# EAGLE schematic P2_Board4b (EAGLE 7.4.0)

## Sheet 1 of 4: Propeller
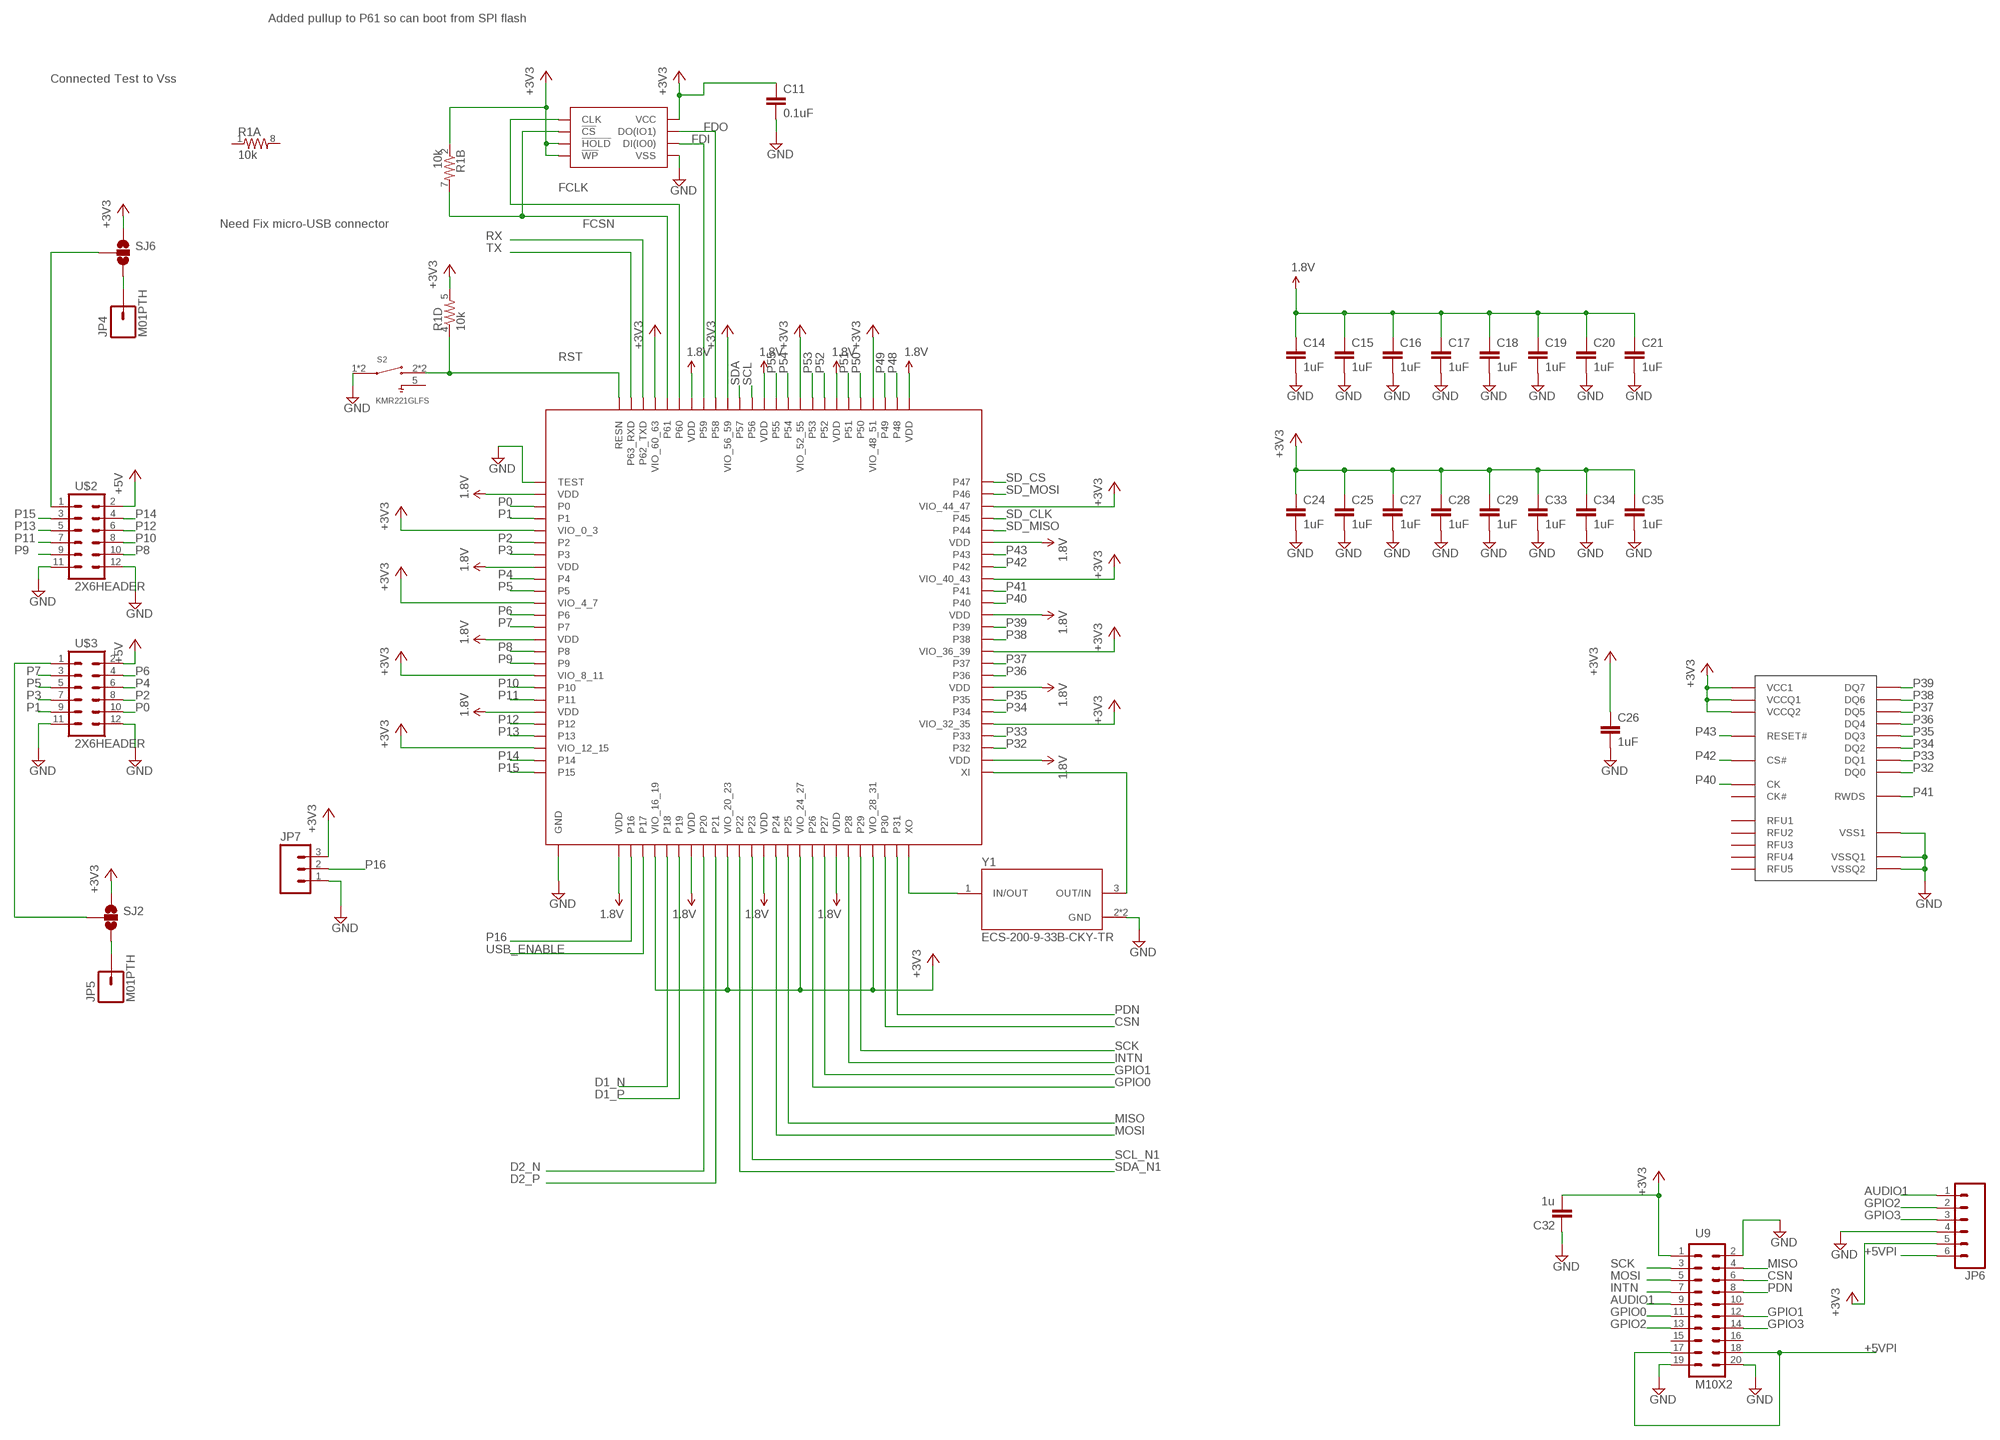
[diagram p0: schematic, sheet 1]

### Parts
C11  0.1uF  1.0UF-25V-+80/-20(0805)  [0805]
C14  1uF  22UF-6.3V-20%(0805)  [0805]
C15  1uF  22UF-6.3V-20%(0805)  [0805]
C16  1uF  22UF-6.3V-20%(0805)  [0805]
C17  1uF  22UF-6.3V-20%(0805)  [0805]
C18  1uF  22UF-6.3V-20%(0805)  [0805]
C19  1uF  22UF-6.3V-20%(0805)  [0805]
C20  1uF  22UF-6.3V-20%(0805)  [0805]
C21  1uF  22UF-6.3V-20%(0805)  [0805]
C24  1uF  22UF-6.3V-20%(0805)  [0805]
C25  1uF  22UF-6.3V-20%(0805)  [0805]
C26  1uF  22UF-6.3V-20%(0805)  [0805]
C27  1uF  22UF-6.3V-20%(0805)  [0805]
C28  1uF  22UF-6.3V-20%(0805)  [0805]
C29  1uF  22UF-6.3V-20%(0805)  [0805]
C32  1u  C-EUC0805  [C0805]
C33  1uF  22UF-6.3V-20%(0805)  [0805]
C34  1uF  22UF-6.3V-20%(0805)  [0805]
C35  1uF  22UF-6.3V-20%(0805)  [0805]
JP4  M01PTH  [1X01]
JP5  M01PTH  [1X01]
JP6  M06LONGPADS  [1X06_LONGPADS]
JP7  M03LONGPADS  [1X03_LONGPADS]
R1  10k  RESISTOR-ARRAY0603-ARV  [0603-ARV]
S2  KMR221GLFS  [SW_KMR221GLFS]
SJ2  SOLDERJUMPER_2WAYPASTE1&2  [SJ_3_PASTE1&2]
SJ6  SOLDERJUMPER_2WAYPASTE1&2  [SJ_3_PASTE1&2]
U2  Propeller 2 - ES  P2X8C4M64P-ES_  [PROPELLER_2]
U3  SPI Flash 16MB (128Mb)  604-10047_:_IC_FLASH_128M_SPI_133MHZ_8SOIC  [SOIC_8_WIDE]
U5  HYPERRAM  [TFBGA24]
U9  M10X2  [2X10]
U$2  2X6HEADER  [6X2HEADER]
U$3  2X6HEADER  [6X2HEADER]
Y1  ECS-200-9-33B-CKY-TR  [XTAL_ECS-200-9-33B-CKY-TR]

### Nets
1.8V: C14.1 C15.1 C16.1 C17.1 C18.1 C19.1 C20.1 C21.1 U2.2(VDD) U2.8(VDD) U2.14(VDD) U2.20(VDD) U2.26(VDD) U2.32(VDD) U2.38(VDD) U2.44(VDD) U2.52(VDD) U2.58(VDD) U2.64(VDD) U2.70(VDD) U2.76(VDD) U2.82(VDD) U2.88(VDD) U2.94(VDD) ; also sheet 4
+3V3: C11.1 C24.1 C25.1 C26.1 C27.1 C28.1 C29.1 C32.2 C33.1 C34.1 C35.1 JP6.5 JP7.3 R1.2 R1.5 SJ2.1 SJ6.1 U2.5(VIO_0_3) U2.11(VIO_4_7) U2.17(VIO_8_11) U2.23(VIO_12_15) U2.29(VIO_16_19) U2.35(VIO_20_23) U2.41(VIO_24_27) U2.47(VIO_28_31) U2.55(VIO_32_35) U2.61(VIO_36_39) U2.67(VIO_40_43) U2.73(VIO_44_47) U2.79(VIO_48_51) U2.85(VIO_52_55) U2.91(VIO_56_59) U2.97(VIO_60_63) U3.3(!WP) U3.7(!HOLD) U3.8(VCC) U5.P$9(VCC1) U5.P$16(VCCQ1) U5.P$24(VCCQ2) U9.1 ; also sheet 3,4
+5V: U$2.2 U$3.2 ; also sheet 2,3,4
+5VPI: JP6.6 U9.17 U9.18 ; also sheet 4
AUDIO1: JP6.1 U9.9
CSN: U2.48(P30) U9.6
D1_N: U2.30(P18) ; also sheet 3
D1_P: U2.31(P19) ; also sheet 3
D2_N: U2.33(P20) ; also sheet 3
D2_P: U2.34(P21) ; also sheet 3
FCLK: U2.95(P60) U3.6(CLK)
FCSN: R1.7 U2.96(P61) U3.1(!CS)
FDI: U2.93(P59) U3.5(DI(IO0))
FDO: U2.92(P58) U3.2(DO(IO1))
GND [power]: C11.2 C14.2 C15.2 C16.2 C17.2 C18.2 C19.2 C20.2 C21.2 C24.2 C25.2 C26.2 C27.2 C28.2 C29.2 C32.1 C33.2 C34.2 C35.2 JP6.4 JP7.1 S2.1 S2.4 U2.1(TEST) U2.EP(GND) U3.4(VSS) U5.P$8(VSS1) U5.P$11(VSSQ1) U5.P$25(VSSQ2) U9.2 U9.19 U9.20 U$2.11 U$2.12 U$3.11 U$3.12 Y1.2(GND) Y1.4(GND) ; also sheet 2,3,4
GPIO0: U2.42(P26) U9.11
GPIO1: U2.43(P27) U9.12
GPIO2: JP6.2 U9.13
GPIO3: JP6.3 U9.14
INTN: U2.45(P28) U9.7
MISO: U2.40(P25) U9.4
MOSI: U2.39(P24) U9.5
N$1: U2.51(XI) Y1.3(OUT/IN)
N$3: U2.50(XO) Y1.1(IN/OUT)
N$10: SJ6.2 U$2.1
N$14: JP4.1 SJ6.3
N$32: SJ2.2 U$3.1
N$33: JP5.1 SJ2.3
P0: U2.3(P0) U$3.10
P1: U2.4(P1) U$3.9
P2: U2.6(P2) U$3.8
P3: U2.7(P3) U$3.7
P4: U2.9(P4) U$3.6
P5: U2.10(P5) U$3.5
P6: U2.12(P6) U$3.4
P7: U2.13(P7) U$3.3
P8: U2.15(P8) U$2.10
P9: U2.16(P9) U$2.9
P10: U2.18(P10) U$2.8
P11: U2.19(P11) U$2.7
P12: U2.21(P12) U$2.6
P13: U2.22(P13) U$2.5
P14: U2.24(P14) U$2.4
P15: U2.25(P15) U$2.3
P16: JP7.2 U2.27(P16) ; also sheet 3
P32: U2.53(P32) U5.P$18(DQ0)
P33: U2.54(P33) U5.P$17(DQ1)
P34: U2.56(P34) U5.P$14(DQ2)
P35: U2.57(P35) U5.P$19(DQ3)
P36: U2.59(P36) U5.P$20(DQ4)
P37: U2.60(P37) U5.P$23(DQ5)
P38: U2.62(P38) U5.P$22(DQ6)
P39: U2.63(P39) U5.P$21(DQ7)
P40: U2.65(P40) U5.P$7(CK)
P41: U2.66(P41) U5.P$13(RWDS)
P42: U2.68(P42) U5.P$3(CS#)
P43: U2.69(P43) U5.P$4(RESET#)
P48: U2.77(P48) ; also sheet 3
P49: U2.78(P49) ; also sheet 3
P50: U2.80(P50) ; also sheet 3
P51: U2.81(P51) ; also sheet 3
P52: U2.83(P52) ; also sheet 3
P53: U2.84(P53) ; also sheet 3
P54: U2.86(P54) ; also sheet 3
P55: U2.87(P55) ; also sheet 3
PDN: U2.49(P31) U9.8
RST: R1.4 S2.2 S2.3 U2.100(RESN) ; also sheet 2,4
RX: U2.98(P62_TXD) ; also sheet 2
SCK: U2.46(P29) U9.3
SCL: U2.89(P56) ; also sheet 3
SCL_N1: U2.37(P23) ; also sheet 3
SD_CLK: U2.72(P45) ; also sheet 3
SD_CS: U2.75(P47) ; also sheet 3
SD_MISO: U2.71(P44) ; also sheet 3
SD_MOSI: U2.74(P46) ; also sheet 3
SDA: U2.90(P57) ; also sheet 3
SDA_N1: U2.36(P22) ; also sheet 3
TX: U2.99(P63_RXD) ; also sheet 2
USB_ENABLE: U2.28(P17) ; also sheet 3
Unconnected: R1.1 R1.8 S2.5 U5.P$2(RFU1) U5.P$5(RFU2) U5.P$6(CK#) U5.P$10(RFU3) U5.P$12(RFU4) U5.P$15(RFU5) U9.10 U9.15 U9.16

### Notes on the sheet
- Added pullup to P61 so can boot from SPI flash
- Connected Test to Vss
- Need Fix micro-USB connector

## Sheet 2 of 4: FT231X
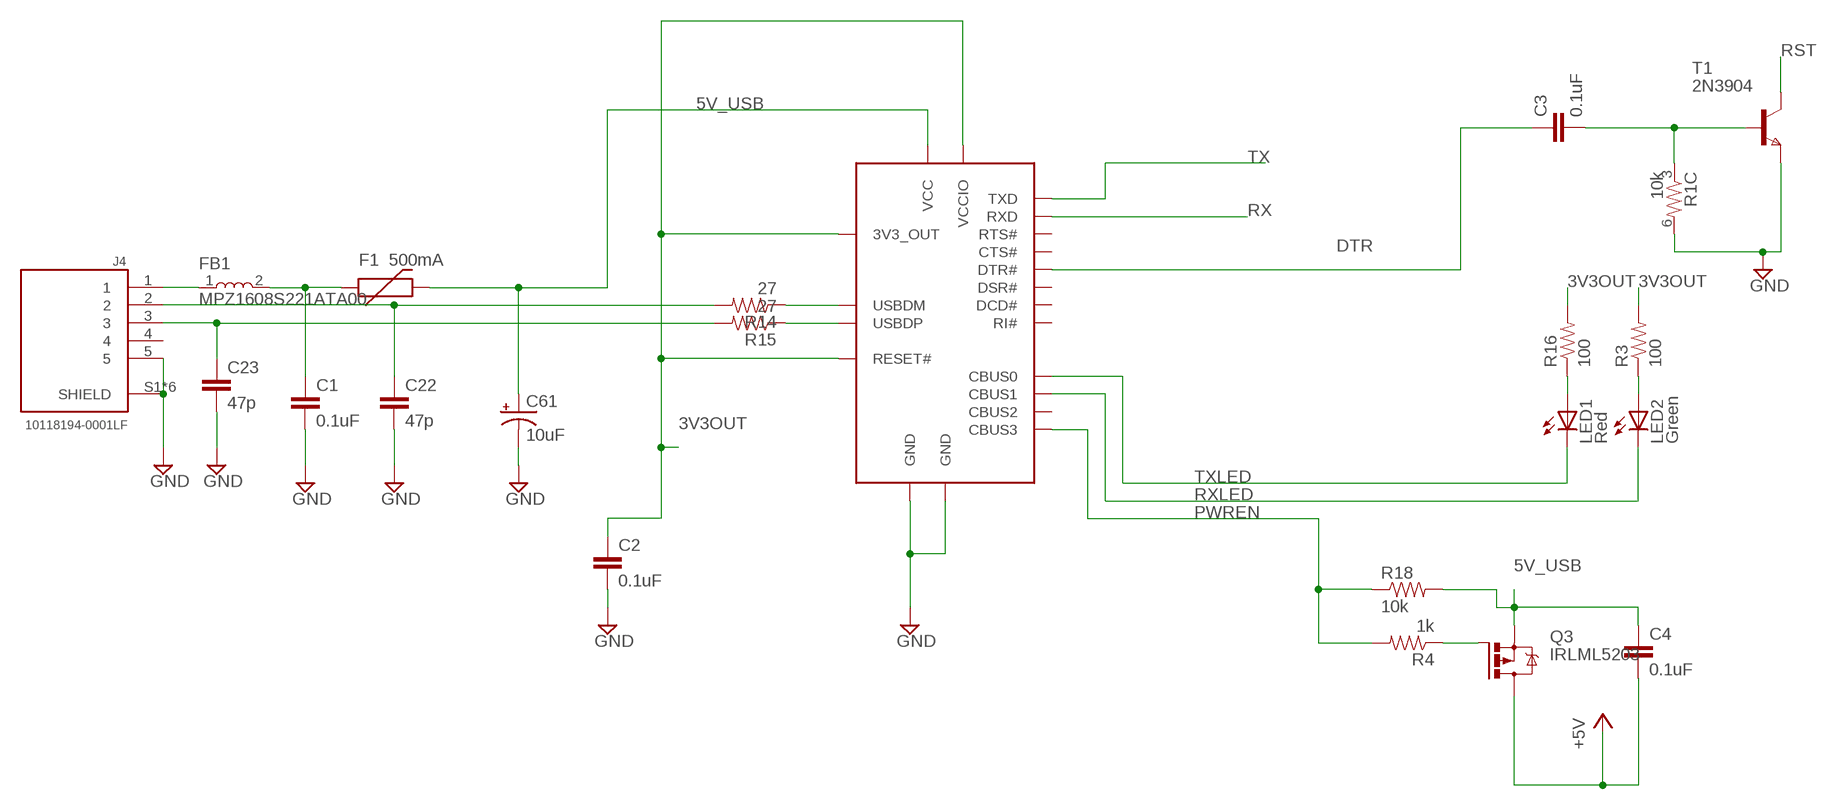
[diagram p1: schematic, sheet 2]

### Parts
C1  0.1uF  1.0UF-25V-+80/-20(0805)  [0805]
C2  0.1uF  1.0UF-25V-+80/-20(0805)  [0805]
C3  0.1uF  1.0UF-25V-+80/-20(0805)  [0805]
C4  0.1uF  1.0UF-25V-+80/-20(0805)  [0805]
C22  47p  1.0UF-25V-+80/-20(0805)  [0805]
C23  47p  1.0UF-25V-+80/-20(0805)  [0805]
C61  10uF  CAP_POL1206  [EIA3216]
F1  500mA  PTCSMD  [PTC-1206]
FB1  MPZ1608S221ATA00  [INDC1608X80]
J4  10118194-0001LF  [AMPHENOL_10118194-0001LF]
LED1  Red  LEDSML0805  [SML0805]
LED2  Green  LEDSML0805  [SML0805]
Q3  IRLML5203  [MICRO3]
R3  100  0.75OHM1/4W1%(0805)  [0805]
R4  1k  0.75OHM1/4W1%(0805)  [0805]
R14  27  0.75OHM1/4W1%(0805)  [0805]
R15  27  0.75OHM1/4W1%(0805)  [0805]
R16  100  0.75OHM1/4W1%(0805)  [0805]
R18  10k  0.75OHM1/4W1%(0805)  [0805]
T1  2N3904  NPNSOT23  [SOT-23]
U1  FT231XS-R  604-00065_:_IC-FTDI,_FT231X  [SSOP20]

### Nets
3V3OUT [power]: C2.1 R3.2 R16.2 U1.3(VCCIO) U1.13(3V3_OUT) U1.14(RESET#)
5V_USB [power]: C4.1 C61.A(+) F1.2 Q3.2(S) R18.2 U1.15(VCC)
+5V: C4.2 Q3.3(D) ; also sheet 1,3,4
DTR: C3.1 U1.1(DTR#)
GND [power]: C1.2 C2.2 C22.2 C23.2 C61.C(-) J4.5 J4.S1(SHIELD) J4.S2(SHIELD) J4.S3(SHIELD) J4.S4(SHIELD) J4.S5(SHIELD) J4.S6(SHIELD) R1.6 T1.2(E) U1.6(GND) U1.16(GND) ; also sheet 1,3,4
N$2: LED1.A R16.1
N$8: FB1.1 J4.1
N$9: C1.1 F1.1 FB1.2
N$11: R14.1 U1.12(USBDM)
N$12: R15.1 U1.11(USBDP)
N$15: C22.1 J4.2 R14.2
N$16: C23.1 J4.3 R15.2
N$18: LED2.A R3.1
N$24: Q3.1(G) R4.1
N$25: C3.2 R1.3 T1.3(B)
PWREN: R4.2 R18.1 U1.19(CBUS3)
RST: T1.1(C) ; also sheet 1,4
RX: U1.4(RXD) ; also sheet 1
RXLED: LED2.C U1.17(CBUS1)
TX: U1.20(TXD) ; also sheet 1
TXLED: LED1.C U1.18(CBUS0)
Unconnected: J4.4 U1.2(RTS#) U1.5(RI#) U1.7(DSR#) U1.8(DCD#) U1.9(CTS#) U1.10(CBUS2)

## Sheet 3 of 4: Wings
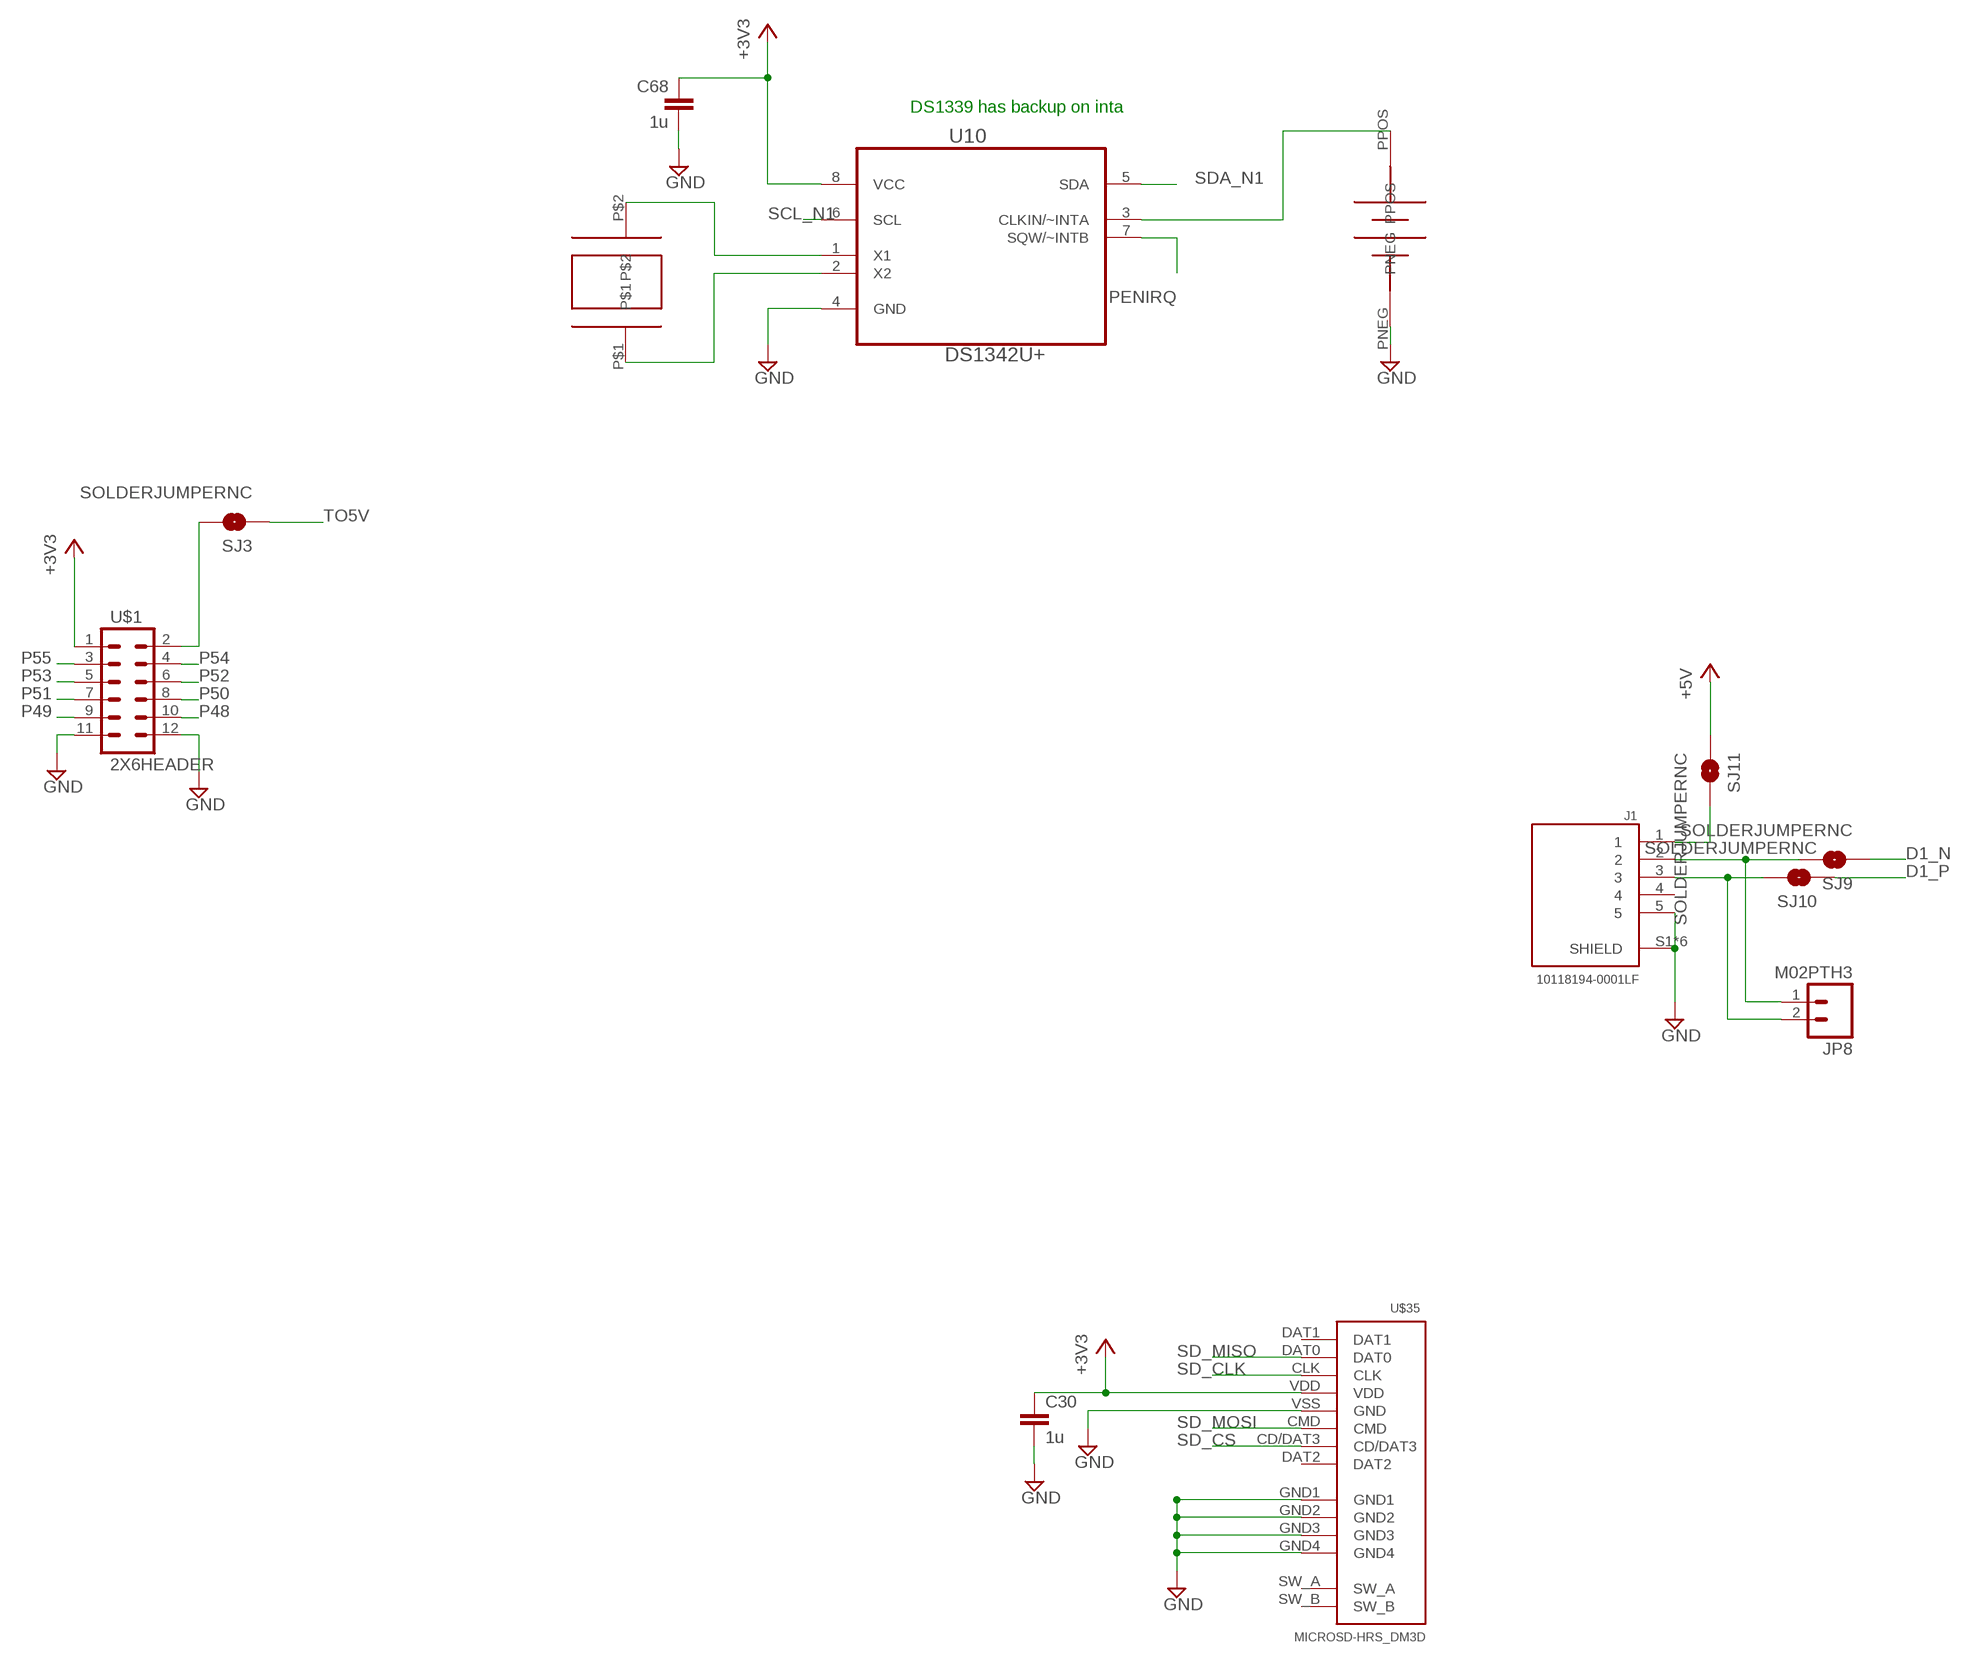
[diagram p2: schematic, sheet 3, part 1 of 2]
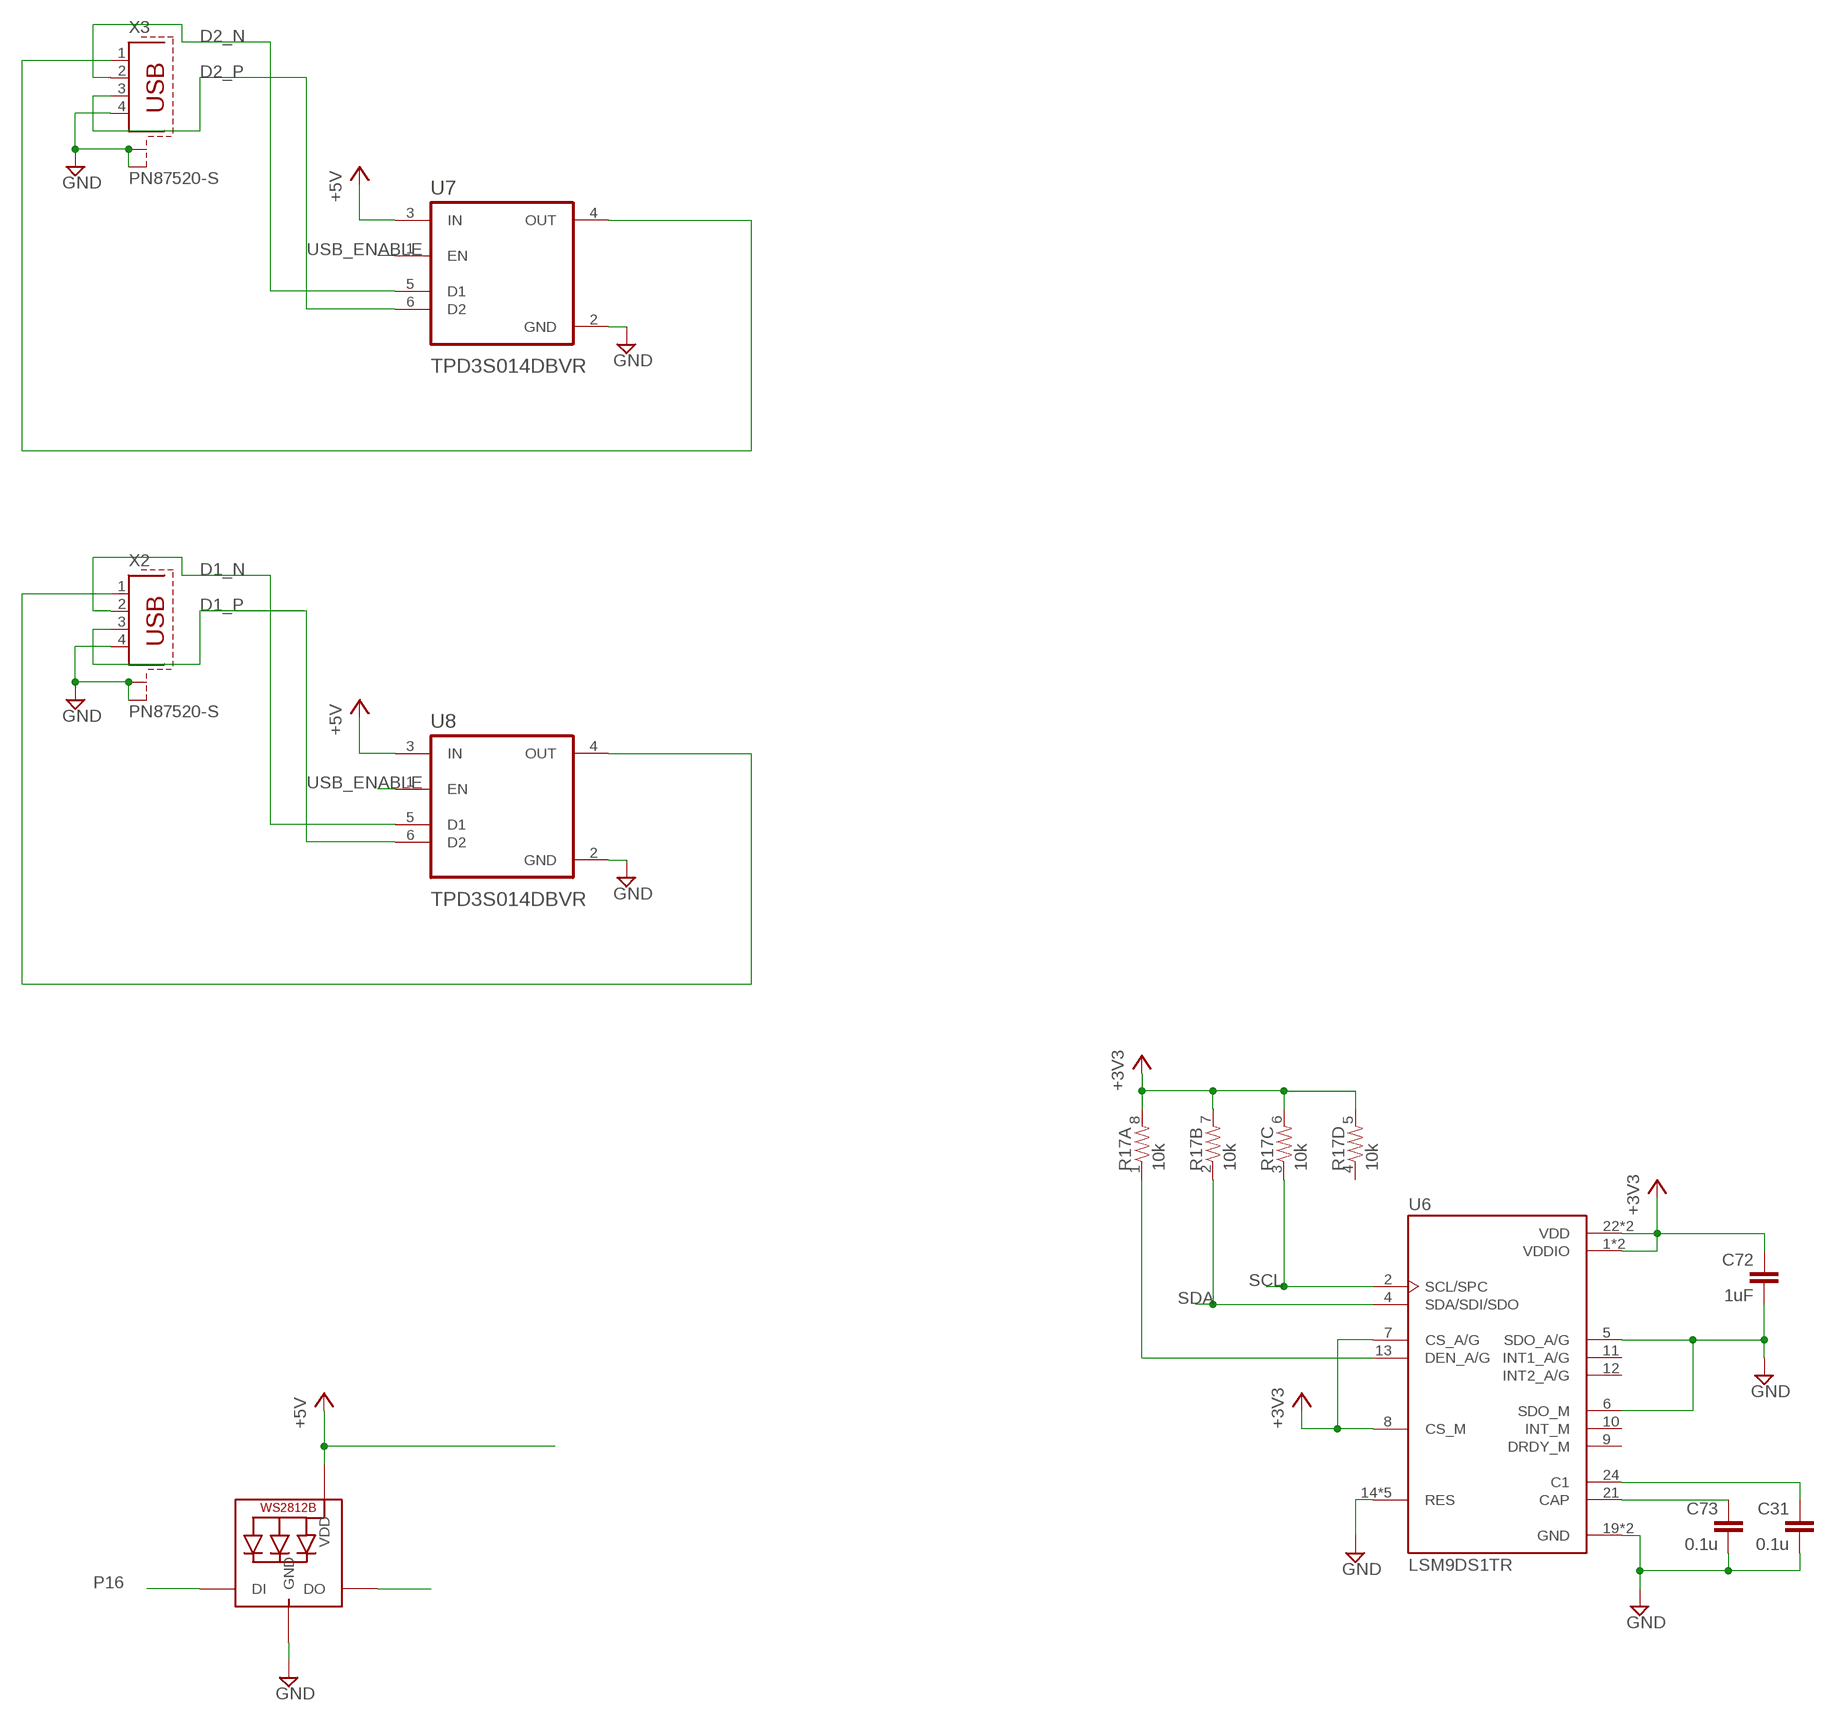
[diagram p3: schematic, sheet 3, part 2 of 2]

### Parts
C30  1u  C-EUC0805  [C0805]
C31  0.1u  4.7UF-6.3V-10%(0603)0603  [0603-CAP]
C68  1u  4.7UF-6.3V-10%(0603)0603  [0603-CAP]
C71  RAY2_SUPERCAP  [RAY2_SUPERCAP]
C72  1uF  4.7UF-6.3V-10%(0603)0603  [0603-CAP]
C73  0.1u  4.7UF-6.3V-10%(0603)0603  [0603-CAP]
J1  10118194-0001LF  [AMPHENOL_10118194-0001LF]
JP8  M02PTH3  [1X02_LONGPADS]
LED3  WS2812B3535  [LED3535]
R17  10k  RESISTOR-ARRAY0603-ARV  [0603-ARV]
SJ3  SOLDERJUMPERNC  [SJ_2S]
SJ9  SOLDERJUMPERNC  [SJ_2S]
SJ10  SOLDERJUMPERNC  [SJ_2S]
SJ11  SOLDERJUMPERNC  [SJ_2S]
U6  LSM9DS1TR  [PQFN43P300X350X102-24N]
U7  TPD3S014DBVR  [SOT95P280X145-6N]
U8  TPD3S014DBVR  [SOT95P280X145-6N]
U10  DS1342U+  [SOP65P490X110-8N]
U$1  2X6HEADER  [6X2HEADER]
U$35  MICROSD-HRS_DM3D  [DM3D]
X2  PN87520-S  [PN87520-S]
X3  PN87520-S  [PN87520-S]
X5  RAY2_SMT_CRYSTAL  [RAY2_SMT_CRYSTAL]

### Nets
+3V3: C30.1 C68.1 C72.1 R17.5 R17.6 R17.7 R17.8 U6.1(VDDIO) U6.3(VDDIO) U6.7(CS_A/G) U6.8(CS_M) U6.22(VDD) U6.23(VDD) U10.8(VCC) U$1.1 U$35.VDD ; also sheet 1,4
+5V: LED3.2(VDD) SJ11.1 U7.3(IN) U8.3(IN) ; also sheet 1,2,4
D1_N: SJ9.1 U8.5(D1) X2.2 ; also sheet 1
D1_P: SJ10.1 U8.6(D2) X2.3 ; also sheet 1
D2_N: U7.5(D1) X3.2 ; also sheet 1
D2_P: U7.6(D2) X3.3 ; also sheet 1
GND [power]: C30.2 C31.2 C68.2 C71.PNEG C72.2 C73.2 J1.5 J1.S1(SHIELD) J1.S2(SHIELD) J1.S3(SHIELD) J1.S4(SHIELD) J1.S5(SHIELD) J1.S6(SHIELD) LED3.4(GND) U6.5(SDO_A/G) U6.6(SDO_M) U6.14(RES) U6.15(RES) U6.16(RES) U6.17(RES) U6.18(RES) U6.19(GND) U6.20(GND) U7.2(GND) U8.2(GND) U10.4(GND) U$1.11 U$1.12 U$35.GND1 U$35.GND2 U$35.GND3 U$35.GND4 U$35.VSS(GND) X2.4 X2.S1 X2.S2 X3.4 X3.S1 X3.S2 ; also sheet 1,2,4
N$17: U7.4(OUT) X3.1
N$28: U8.4(OUT) X2.1
N$29: C73.1 U6.21(CAP)
N$30: C31.1 U6.24(C1)
N$31: R17.1 U6.13(DEN_A/G)
N$39: LED3.3(DO)
N$40: J1.2 JP8.1 SJ9.2
N$41: J1.3 JP8.2 SJ10.2
N$42: J1.1 SJ11.2
N$43: SJ3.2 U$1.2
N$78: C71.PPOS U10.3(CLKIN/~INTA)
N$79: U10.2(X2) X5.P$1
N$81: U10.1(X1) X5.P$2
P16: LED3.1(DI) ; also sheet 1
P48: U$1.10 ; also sheet 1
P49: U$1.9 ; also sheet 1
P50: U$1.8 ; also sheet 1
P51: U$1.7 ; also sheet 1
P52: U$1.6 ; also sheet 1
P53: U$1.5 ; also sheet 1
P54: U$1.4 ; also sheet 1
P55: U$1.3 ; also sheet 1
PENIRQ: U10.7(SQW/~INTB)
SCL: R17.3 U6.2(SCL/SPC) ; also sheet 1
SCL_N1: U10.6(SCL) ; also sheet 1
SD_CLK: U$35.CLK ; also sheet 1
SD_CS: U$35.CD/DAT3 ; also sheet 1
SD_MISO: U$35.DAT0 ; also sheet 1
SD_MOSI: U$35.CMD ; also sheet 1
SDA: R17.2 U6.4(SDA/SDI/SDO) ; also sheet 1
SDA_N1: U10.5(SDA) ; also sheet 1
TO5V: SJ3.1 ; also sheet 4
USB_ENABLE: U7.1(EN) U8.1(EN) ; also sheet 1
Unconnected: J1.4 R17.4 U6.9(DRDY_M) U6.10(INT_M) U6.11(INT1_A/G) U6.12(INT2_A/G) U$35.DAT1 U$35.DAT2 U$35.SW_A U$35.SW_B

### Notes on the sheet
- DS1339 has backup on inta

## Sheet 4 of 4: Power
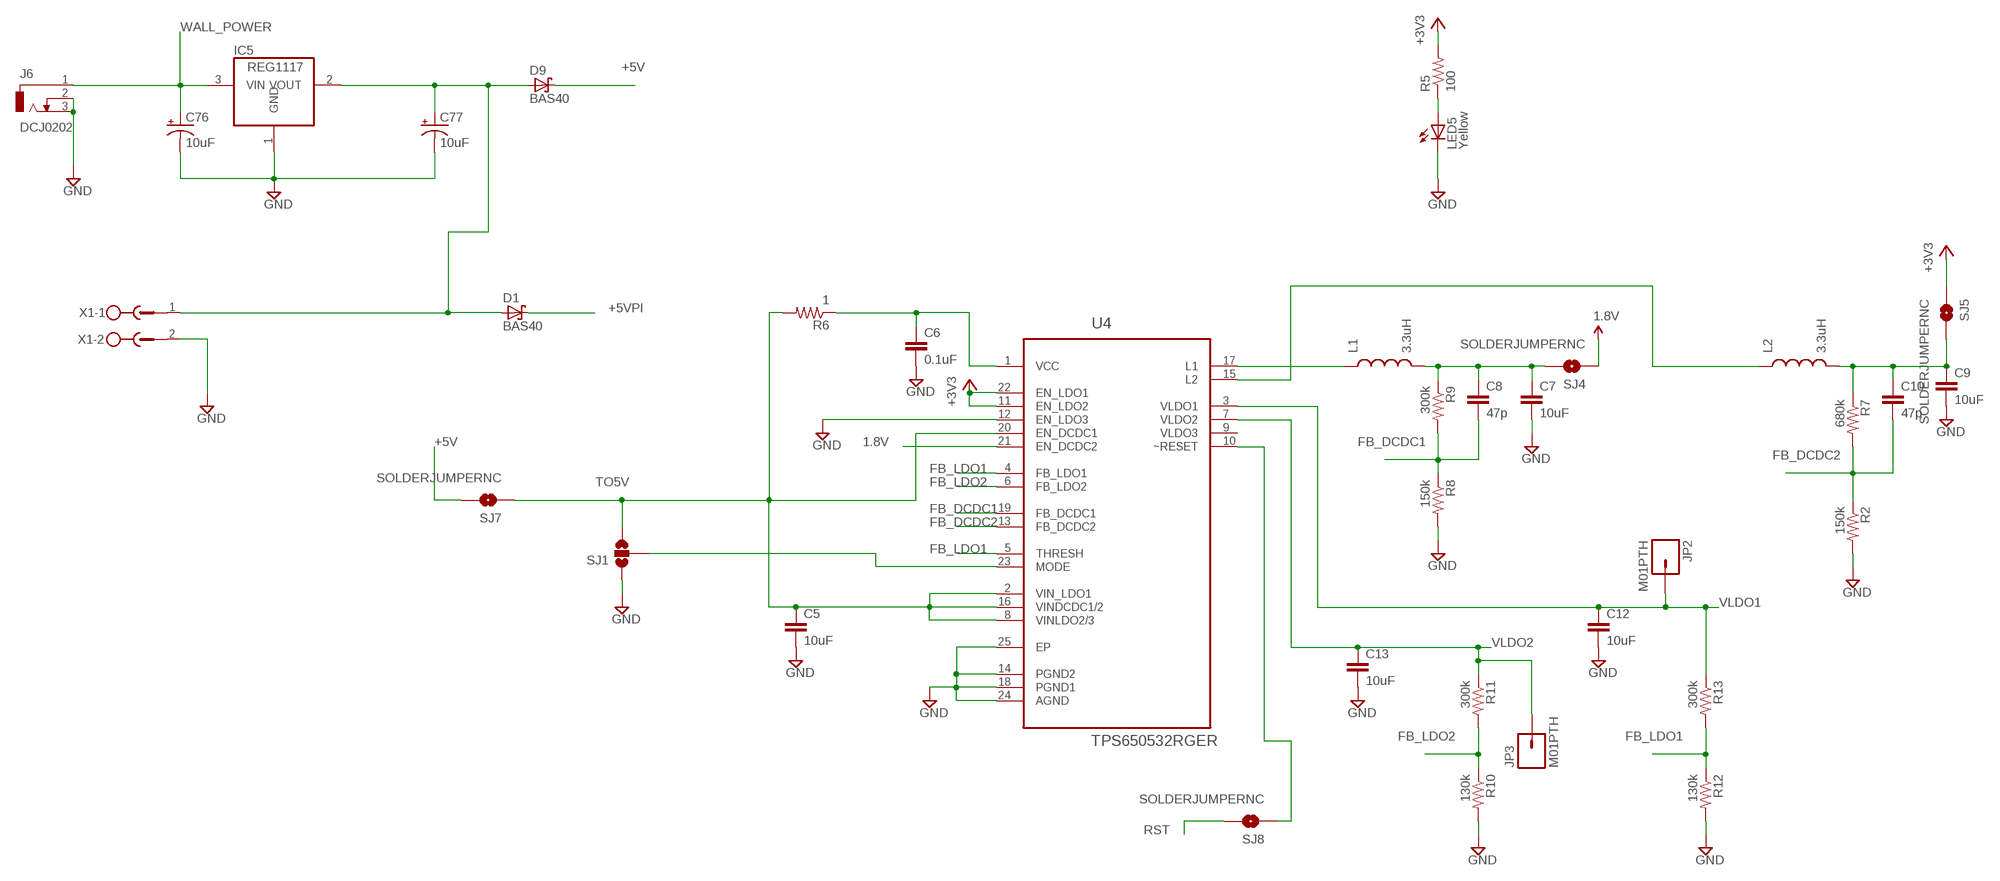
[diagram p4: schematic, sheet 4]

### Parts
C5  10uF  22UF-6.3V-20%(0805)  [0805]
C6  0.1uF  1.0UF-25V-+80/-20(0805)  [0805]
C7  10uF  22UF-6.3V-20%(0805)  [0805]
C8  47p  1.0UF-25V-+80/-20(0805)  [0805]
C9  10uF  22UF-6.3V-20%(0805)  [0805]
C10  47p  1.0UF-25V-+80/-20(0805)  [0805]
C12  10uF  22UF-6.3V-20%(0805)  [0805]
C13  10uF  22UF-6.3V-20%(0805)  [0805]
C76  10uF  10UF-16V-10%(TANT)  [EIA3216]
C77  10uF  10UF-16V-10%(TANT)  [EIA3216]
D1  BAS40  [SOT23]
D9  BAS40  [SOT23]
IC5  REG1117  [SOT223]
J6  DCJ0202  [DCJ0202]
JP2  M01PTH  [1X01]
JP3  M01PTH  [1X01]
L1  3.3uH  INDUCTOR1210  [1210]
L2  3.3uH  INDUCTOR1210  [1210]
LED5  Yellow  LEDSML0805  [SML0805]
R2  150k  0.75OHM1/4W1%(0805)  [0805]
R5  100  0.75OHM1/4W1%(0805)  [0805]
R6  1  0.75OHM1/4W1%(0805)  [0805]
R7  680k  0.75OHM1/4W1%(0805)  [0805]
R8  150k  0.75OHM1/4W1%(0805)  [0805]
R9  300k  0.75OHM1/4W1%(0805)  [0805]
R10  130k  0.75OHM1/4W1%(0805)  [0805]
R11  300k  0.75OHM1/4W1%(0805)  [0805]
R12  130k  0.75OHM1/4W1%(0805)  [0805]
R13  300k  0.75OHM1/4W1%(0805)  [0805]
SJ1  SOLDERJUMPER_2WAYPASTE1&2  [SJ_3_PASTE1&2]
SJ4  SOLDERJUMPERNC  [SJ_2S]
SJ5  SOLDERJUMPERNC  [SJ_2S]
SJ7  SOLDERJUMPERNC  [SJ_2S]
SJ8  SOLDERJUMPERNC  [SJ_2S]
U4  TPS650532RGER  [QFN50P400X400X100-25N]
X1  MSTBV2  [MSTBV2]

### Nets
1.8V: SJ4.1 U4.21(EN_DCDC2) ; also sheet 1
+3V3: R5.2 SJ5.1 U4.11(EN_LDO2) U4.22(EN_LDO1) ; also sheet 1,3
+5_VIN: C77.A(+) D1.1(A) D9.1(A) IC5.2(VOUT) X1.1
+5V: D9.3(C) SJ7.2 ; also sheet 1,2,3
+5VPI: D1.3(C) ; also sheet 1
FB_DCDC1: C8.2 R8.1 R9.2 U4.19(FB_DCDC1)
FB_DCDC2: C10.2 R2.1 R7.2 U4.13(FB_DCDC2)
FB_LDO1: R12.1 R13.2 U4.4(FB_LDO1) U4.5(THRESH)
FB_LDO2: R10.1 R11.2 U4.6(FB_LDO2)
GND [power]: C5.2 C6.2 C7.2 C9.2 C12.2 C13.2 C76.C(-) C77.C(-) IC5.1(GND) J6.2 J6.3 LED5.C R2.2 R8.2 R10.2 R12.2 SJ1.1 U4.12(EN_LDO3) U4.14(PGND2) U4.18(PGND1) U4.24(AGND) U4.25(EP) X1.2 ; also sheet 1,2,3
N$4: L2.1 U4.15(L2)
N$5: SJ1.2 U4.23(MODE)
N$6: C6.1 R6.1 U4.1(VCC)
N$7: L1.1 U4.17(L1)
N$13: SJ8.1 U4.10(~RESET)
N$22: C7.1 C8.1 L1.2 R9.1 SJ4.2
N$34: C9.1 C10.1 L2.2 R7.1 SJ5.2
N$45: LED5.A R5.1
RST: SJ8.2 ; also sheet 1,2
TO5V: C5.1 R6.2 SJ1.3 SJ7.1 U4.2(VIN_LDO1) U4.8(VINLDO2/3) U4.16(VINDCDC1/2) U4.20(EN_DCDC1) ; also sheet 3
VLDO1: C12.1 JP2.1 R13.1 U4.3(VLDO1)
VLDO2: C13.1 JP3.1 R11.1 U4.7(VLDO2)
WALL_POWER: C76.A(+) IC5.3(VIN) J6.1
Unconnected: U4.9(VLDO3)

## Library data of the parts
C1-C4 C6 C8 C10 C11 C22 C23 = SparkFun-Capacitors:1.0UF-25V-+80/-20(0805); PROD_ID: CAP-11625; VALUE: 1.0uF
C5 C7 C9 C12-C21 C24-C29 C33-C35 = SparkFun-Capacitors:22UF-6.3V-20%(0805): Ceramic; PROD_ID: CAP-08402; VALUE: 22uF
C30 C32 = rcl:C-EU: CAPACITOR, European symbol
C31 C68 C72 C73 = SparkFun-Capacitors:4.7UF-6.3V-10%(0603): CAP-08280; PROD_ID: CAP-08280; VALUE: 4.7uF
C61 = SparkFun:CAP_POL: Capacitor Polarized
C71 = Manta1:RAY2_SUPERCAP
C76 C77 = SparkFun-Capacitors:10UF-16V-10%(TANT): CAP-00811; PROD_ID: CAP-00811
D1 D9 = diode:BAS40: Silicon Schottky Diodes
F1 = SparkFun:PTC: Resettable Fuse PTC
FB1 = ray2:MPZ1608S221ATA00: Ind Chip Bead Multi-Layer 220Ohm 25% 100MHz Ferrite 2.2A 0603 Punched Paper T/R; DESCRIPTION: Ind Chip Bead Multi-Layer 220Ohm 25% 100MHz Ferrite 2.2A 0603 Punched Paper T/R; DIGI-KEY_PART_NUMBER: 445-1565-1-ND; DIGI-KEY_PURCHASE_URL: https://www.digikey.com/product-detail/en/tdk-corporation/MPZ1608S221ATA00/445-1565-1-ND/571895?utm_source=snapeda&utm_medium=aggregator&utm_campaign=symbol; MF: TDK; MP: MPZ1608S221ATA00; PACKAGE: 0603 TDK
IC5 = burr-brown:REG1117: 800mA and 1A Low Dropout (LDO) Positive Regulator 1.8V, 2.5V, 2.85V, 3.3V, 5V, and Adj; MPN: REG1117; OC_FARNELL: 1097566; OC_NEWARK: 14P6981
J1 J4 = ray2:10118194-0001LF: Micro Usb, 2.0 Type b, Rcpt, Smt; DESCRIPTION: Micro Usb, 2.0 Type b, Rcpt, Smt; DIGI-KEY_PART_NUMBER: 609-4618-1-ND; DIGI-KEY_PURCHASE_URL: https://www.digikey.com/product-detail/en/amphenol-icc-fci/10118194-0001LF/609-4618-1-ND/2785382?utm_source=snapeda&utm_medium=aggregator&utm_campaign=symbol; MF: Amphenol ICC; MP: 10118194-0001LF; PACKAGE: None
J6 = con-jack:DCJ0202: DC POWER JACK Source: DCJ0202.pdf; OC_FARNELL: unknown; OC_NEWARK: unknown
JP2-JP5 = SparkFun-Connectors:M01: Header 1
JP6 = SparkFun-Connectors:M06: Header 6 Standard 6-pin 0.1" header. Use with straight break away headers (SKU : PRT-00116), right angle break away headers (PRT-00553), swiss pins (PRT-00743), machine pins (PRT-00117), and female headers (PRT-00115). Molex polarized connector foot print use with SKU : PRT-08094 with associated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
JP7 = SparkFun-Connectors:M03: Header 3 Standard 3-pin 0.1" header. Use with straight break away headers (SKU : PRT-00116), right angle break away headers (PRT-00553), swiss pins (PRT-00743), machine pins (PRT-00117), and female headers (PRT-00115). Molex polarized connector foot print use with SKU : PRT-08232 with associated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
JP8 = SparkFun-Connectors:M02: Standard 2-pin 0.1" header. Use with
L1 L2 = SparkFun-Passives:INDUCTOR: Inductors
LED1 LED2 LED5 = led:LED: LED
LED3 = adafruit:WS2812B
Q3 = transistor-power:IRLML5203: HEXFET P-Channel Power MOSFET
R1 R17 = SparkFun-Passives:RESISTOR-ARRAY: Array Chip Resistor Source: RS Component / Phycomp
R2-R16 R18 = SparkFun-Resistors:0.75OHM1/4W1%(0805): RES-08474; PROD_ID: RES-08474; VALUE: 0.75
S2 = ray2:KMR221GLFS: Switch Tactile N.O. SPST Button Gull Wing 0.05A 32VDC 1VA 200000Cycles 2N SMD Automotive T/R; DESCRIPTION: Switch Tactile N.O. SPST Button Gull Wing 0.05A 32VDC 1VA 200000Cycles 2N SMD Automotive T/R; DIGI-KEY_PART_NUMBER: 401-1427-1-ND; DIGI-KEY_PURCHASE_URL: https://www.digikey.com/product-detail/en/c-k/KMR221GLFS/401-1427-1-ND/550466?utm_source=snapeda&utm_medium=aggregator&utm_campaign=symbol; MF: C&K; MP: KMR221GLFS; PACKAGE: None
SJ1 SJ2 SJ6 = SparkFun-Passives:SOLDERJUMPER_2WAY: Solder Jumper 2 way solder jumper
SJ3-SJ5 SJ7-SJ11 = SparkFun-Passives:SOLDERJUMPER: Solder Jumper
T1 = zetex:NPNSOT23: NPN TRANSISTOR; MPN: DSS20201L-7; OC_FARNELL: 1710688; OC_NEWARK: 25R4555
U1 = ray2:604-00065_:_IC-FTDI,_FT231X; MANUFACTURER: FTDI : FT231XS-R; POPULATED: True
U2 = ray2:P2X8C4M64P-ES_; MANUFACTURER: Parallax : P2X8C4M64P-ES
U3 = ray2:604-10047_:_IC_FLASH_128M_SPI_133MHZ_8SOIC; MANUFACTURER: Winbond : W25Q128JVSIM TR
U4 = ray2:TPS650532RGER: 5-CHANNEL POWER MGMT IC WITH TWO STEP DOWN CONVERTERS; DESCRIPTION: 5-Channel Power Management IC _PMIC_ with two step down converters and 3 low-input voltage LDOs 24-VQFN -40 to 85; DIGI-KEY_PART_NUMBER: 296-25183-1-ND; DIGI-KEY_PURCHASE_URL: https://www.digikey.com/product-detail/en/texas-instruments/TPS650532RGER/296-25183-1-ND/2171110?utm_source=snapeda&utm_medium=aggregator&utm_campaign=symbol; MF: Texas Instruments; MP: TPS650532RGER; PACKAGE: VQFN-24 Texas Instruments
U5 = ray2:HYPERRAM: ISSI HyperRAM with 24-ball BGA
U6 = ray2:LSM9DS1TR: The LSM9DS1 is a system-in-package featuring a 3D digital linear acceleration sensor, a 3D digital angular rate sensor, and a 3D digital magnetic sensor.; DESCRIPTION: LSM9DS1 Series ±2/±4/±8/±16 g 3D Digital Linear Acceleration Sensor - LGA-24; DIGI-KEY_PART_NUMBER: 497-14946-1-ND; DIGI-KEY_PURCHASE_URL: https://www.digikey.com/product-detail/en/stmicroelectronics/LSM9DS1TR/497-14946-1-ND/4988079?utm_source=snapeda&utm_medium=aggregator&utm_campaign=symbol; MF: STMicroelectronics; MP: LSM9DS1TR; PACKAGE: TFLGA-24 STMicroelectronics
U7 U8 = ray2:TPD3S014DBVR: Current Limit Switch and D+/D? ESD Protection for USB Host Ports 6-SOT-23 -40 to 85; DESCRIPTION: Current Limit Switch and D+/D? ESD Protection for USB Host Ports 6-SOT-23 -40 to 85; DIGI-KEY_PART_NUMBER: 296-38835-1-ND; DIGI-KEY_PURCHASE_URL: https://www.digikey.com/product-detail/en/texas-instruments/TPD3S014DBVR/296-38835-1-ND/5138398?utm_source=snapeda&utm_medium=aggregator&utm_campaign=symbol; MF: Texas Instruments; MP: TPD3S014DBVR; PACKAGE: SOT-23-6 Texas Instruments
U9 = SparkFun-Connectors:M10X2: This was SPECIALLY designed to be used with our Graphic LCD Backpack. Be sure you want to use this! It is not only staggered on each line of header holes, but IT IS ALSO offset of the center point of the top and bottom lines by 5 mil. This causes the headers to lock into place on the "standard"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
U10 = Maxim_By_element14_Batch_1:DS1342U+: Low-Current I2C RTCs for High-ESR Crystals; MPN: DS1342U+; OC_FARNELL: -; OC_NEWARK: 68R0491; PACKAGE: SOP-8; SUPPLIER: Maxim
U$1-U$3 = ray2:2X6HEADER
U$35 = hrs_DM3D-SF:MICROSD-HRS_DM3D
X1 = con-phoenix-500:MSTBV2: PHOENIX; OC_FARNELL: unknown; OC_NEWARK: unknown
X2 X3 = con-berg:PN87520-S; OC_FARNELL: unknown; OC_NEWARK: unknown
X5 = Manta1:RAY2_SMT_CRYSTAL
Y1 = ray2:ECS-200-9-33B-CKY-TR: The miniature ECS-33B is a compact SMD Crystal. The industry standard 3.2 x 2.5 x 0.8 mm ceramic package is ideal for today’s wireless applications.; DESCRIPTION: CRYSTAL 20MHZ 9PF SMD; DIGI-KEY_PART_NUMBER: XC2464CT-ND; DIGI-KEY_PURCHASE_URL: https://www.digikey.com/product-detail/en/ecs-inc/ECS-200-9-33B-CKY-TR/XC2464CT-ND/8023399?utm_source=snapeda&utm_medium=aggregator&utm_campaign=symbol; MF: ECS Inc.; MP: ECS-200-9-33B-CKY-TR; PACKAGE: SMD-4 ECS Inc.

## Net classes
1 power: width 0.254 mm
